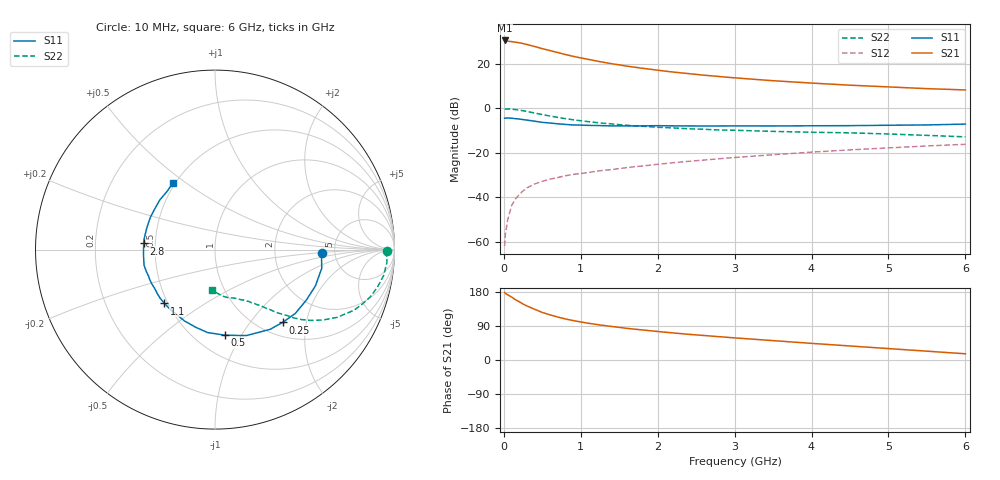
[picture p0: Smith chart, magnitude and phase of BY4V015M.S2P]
! SIEMENS Small Signal Semiconductors
! BFY420
! Si NPN RF SIEGET Grounded Emitter Transistor in MICRO-X
! VCE = 4 V  IC = 15 mA
! Common Emitter S-Parameters:  October  1996
# GHz  S  MA  R  50
!  f  S11  S21  S12  S22
! GHz  MAG  ANG  MAG  ANG  MAG  ANG  MAG  ANG
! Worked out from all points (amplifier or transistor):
!   36 points, 10 MHz to 6 GHz, reference 50 ohm
!   highest |S21| = 30.4 dB at 10 MHz (marker M1)
!   |S21| within 3 dB of that: start of sweep to 430.4 MHz
!   unconditionally stable (mu >= 1): start of sweep to 15.26 MHz; 2.209 GHz to end of sweep
!   at 250 MHz: K = 0.29, MSG = 33.1 dB, |S12| = -37.1 dB
!   at 1.4 GHz: K = 0.85, MSG = 23.8 dB, |S12| = -27.6 dB
!   at 6 GHz: K = 1.07, MAG = 10.6 dB, |S12| = -16.2 dB
!   S11 on the Smith chart (normalised r, x): 10 MHz: 3.93, -0.24; 250 MHz: 1.25, -1.47; 500 MHz: 0.69, -0.85; 1.1 GHz: 0.48, -0.35; 2.8 GHz: 0.43, +0.03; 6 GHz: 0.49, +0.45
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0.01  0.5959 -1.9  33.07 178.3  0.0008 37.3  0.9594 -0.5
0.02  0.5948 -3.8  32.52 175.9  0.0015 70.6  0.9551 -1.4
0.1  0.5949 -19.9  31.23 166.3  0.0065 73.3  0.9503 -8.8
0.15  0.5812 -29.2  30.2 159.1  0.0091 71.8  0.9291 -13.0
0.2  0.5715 -38.5  29.35 153.8  0.0115 71.2  0.9053 -16.8
0.25  0.5537 -47.1  28.14 147.7  0.0139 68.3  0.8733 -20.5
0.3  0.5399 -55.4  26.85 142.6  0.0163 66.1  0.8446 -23.6
0.4  0.5099 -69.9  24.23 133.9  0.0199 62.4  0.7784 -29.0
0.5  0.4803 -83.3  21.65 125.4  0.0228 60.3  0.7185 -33.1
0.6  0.4639 -95.1  19.58 119.2  0.0256 57.7  0.6665 -36.3
0.7  0.4458 -104.0  17.74 113.4  0.0277 57.5  0.6212 -38.9
0.8  0.4322 -113.3  15.99 108.4  0.0304 55.1  0.582 -40.9
0.9  0.4205 -119.9  14.58 104.1  0.0327 54.8  0.5493 -42.2
1.1  0.4113 -133.2  12.44 97.0  0.036 55.4  0.4978 -45.2
1.3  0.4041 -142.7  10.67 91.1  0.0404 55.8  0.4576 -47.2
1.6  0.4003 -155.2  8.775 83.5  0.0462 55.3  0.4129 -50.2
2.2  0.4009 -172.1  6.46 71.5  0.0595 54.8  0.3601 -55.4
2.8  0.3987 175.1  5.13 61.5  0.0733 53.0  0.3236 -60.1
3.5  0.3989 161.9  4.128 51.1  0.0901 49.3  0.3012 -65.4
4.5  0.4052 145.8  3.278 37.0  0.1157 42.5  0.2795 -74.1
5.5  0.4205 129.2  2.742 23.3  0.1419 34.4  0.2451 -86.3
6  0.4394 122.3  2.564 16.4  0.1545 30.0  0.2272 -94.1
